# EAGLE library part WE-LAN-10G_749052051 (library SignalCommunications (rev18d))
WE-LAN 10G Transformer 10Gbit Base-T - Compliant with standards: IEEE 802.3an and upcoming IEEE 802.3bt - SMD -- Ethernet -- Ethernet speed up to 10Gbit/s --Power over Ethernet PoE and PoE+ --10Gbit with ETR and PoE up to 150 W (for industrial applications) Details see: http://katalog.we-online.de/en/pbs/WE-LAN-10G Created By Yingchun,Shan (C) Würth Elektronik
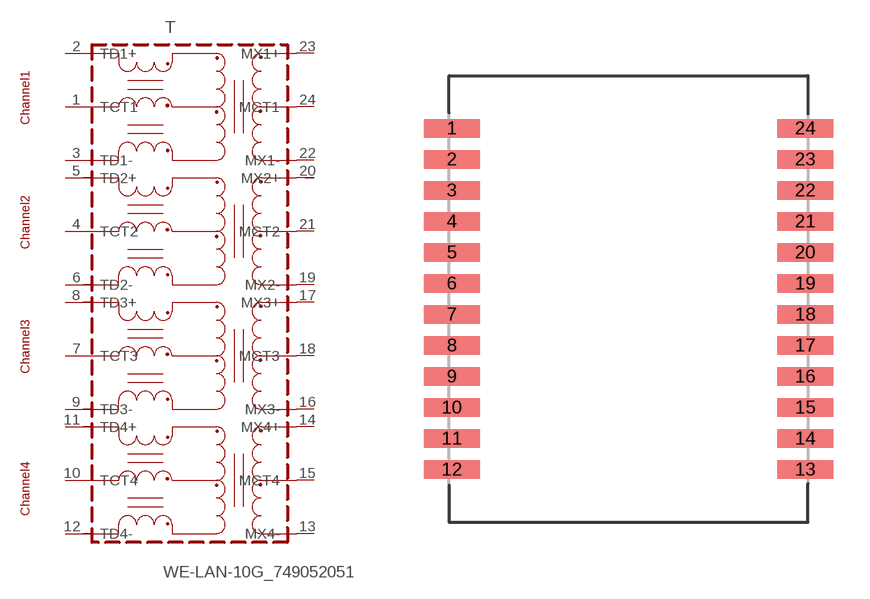
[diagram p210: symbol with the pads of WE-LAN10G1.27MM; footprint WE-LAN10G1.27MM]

Designator prefix T

## WE-LAN-10G_749052051  [WE-LAN10G1.27MM]
1  TCT1
2  TD1+
3  TD1-
4  TCT2
5  TD2+
6  TD2-
7  TCT3
8  TD3+
9  TD3-
10  TCT4
11  TD4+
12  TD4-
13  MX4-
14  MX4+
15  MCT4
16  MX3-
17  MX3+
18  MCT3
19  MX2-
20  MX2+
21  MCT2
22  MX1-
23  MX1+
24  MCT1

## Footprint WE-LAN10G1.27MM (pad centres in mm)
WE-LAN 10G:1.27mm
smd 2.29 x 0.76: 1 -7.24,6.985; 2 -7.24,5.715; 3 -7.24,4.445; 4 -7.24,3.175; 5 -7.24,1.905; 6 -7.24,0.635; 7 -7.24,-0.635; 8 -7.24,-1.905; 9 -7.24,-3.175; 10 -7.24,-4.445; 11 -7.24,-5.715; 12 -7.24,-6.985; 13 7.24,-6.985; 14 7.24,-5.715; 15 7.24,-4.445; 16 7.24,-3.175; 17 7.24,-1.905; 18 7.24,-0.635; 19 7.24,0.635; 20 7.24,1.905; 21 7.24,3.175; 22 7.24,4.445; 23 7.24,5.715; 24 7.24,6.985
